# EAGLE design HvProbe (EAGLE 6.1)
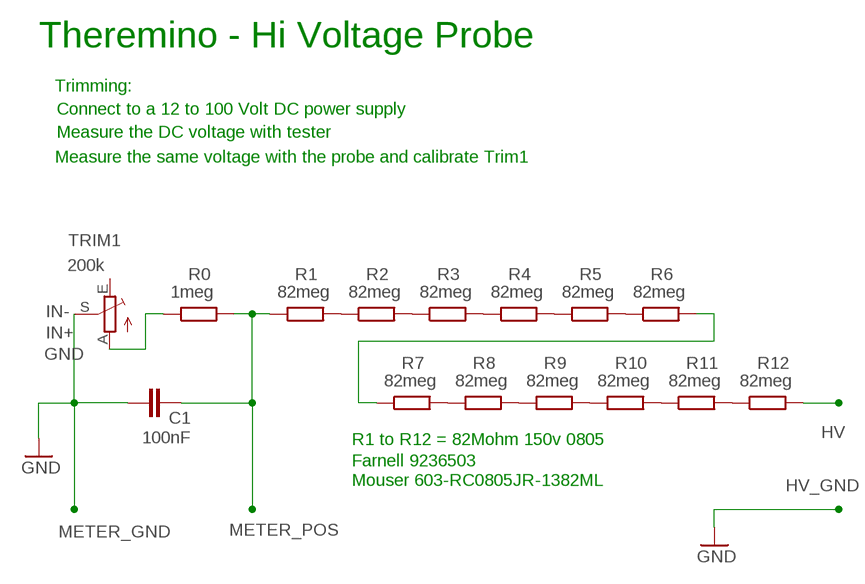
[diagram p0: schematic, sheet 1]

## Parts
C1  100nF  C-EUC0805_L  [C0805_L]
R0  1meg  R-EU_R0805_L  [R0805_L]
R1  82meg  R-EU_R0805_L  [R0805_L]
R2  82meg  R-EU_R0805_L  [R0805_L]
R3  82meg  R-EU_R0805_L  [R0805_L]
R4  82meg  R-EU_R0805_L  [R0805_L]
R5  82meg  R-EU_R0805_L  [R0805_L]
R6  82meg  R-EU_R0805_L  [R0805_L]
R7  82meg  R-EU_R0805_L  [R0805_L]
R8  82meg  R-EU_R0805_L  [R0805_L]
R9  82meg  R-EU_R0805_L  [R0805_L]
R10  82meg  R-EU_R0805_L  [R0805_L]
R11  82meg  R-EU_R0805_L  [R0805_L]
R12  82meg  R-EU_R0805_L  [R0805_L]
TRIM1  200k  TRIMMERTRIM_2H  [TRIM_2H]

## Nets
HV: R12.2
METER_GND: C1.1 TRIM1.S ; supply symbol labelled GND
METER_POS: C1.2 R0.2 R1.1
N$1: R1.2 R2.1
N$2: R2.2 R3.1
N$3: R3.2 R4.1
N$4: R4.2 R5.1
N$5: R5.2 R6.1
N$6: R6.2 R7.1
N$7: R7.2 R8.1
N$8: R8.2 R9.1
N$9: R9.2 R10.1
N$10: R11.2 R12.1
N$11: R10.2 R11.1
N$12: R0.1 TRIM1.A
Unconnected: TRIM1.E

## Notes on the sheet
- Theremino - Hi Voltage Probe
- Trimming:
- Connect to a 12 to 100 Volt DC power supply
- Measure the DC voltage with tester
- Measure the same voltage with the probe and calibrate Trim1
- IN-
- IN+
- GND
- R1 to R12 = 82Mohm 150v 0805
- Farnell 9236503
- Mouser 603-RC0805JR-1382ML

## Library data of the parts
C1 = 00-LIVIO:C-EU: CAPACITOR, European symbol
R0 R1-R12 = 00-LIVIO:R-EU_: RESISTOR, European symbol
TRIM1 = 00-LIVIO:TRIMMER: Horizzontal and Vertical trimmers

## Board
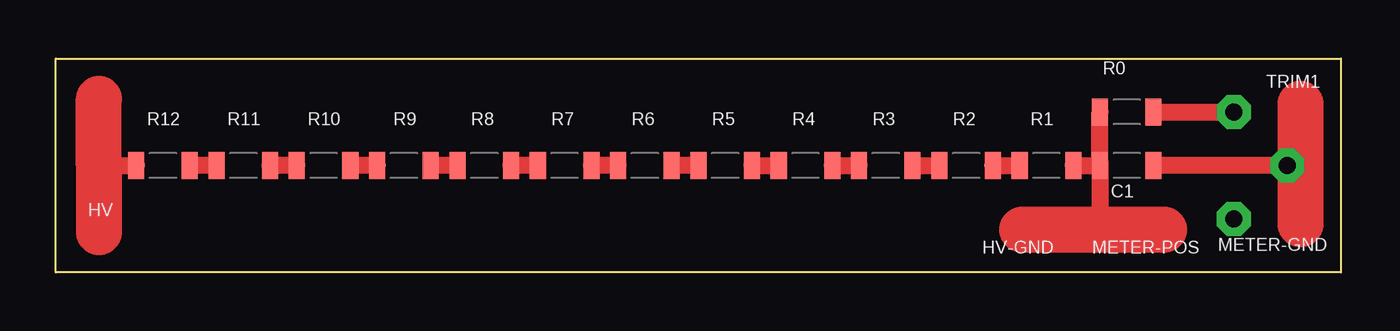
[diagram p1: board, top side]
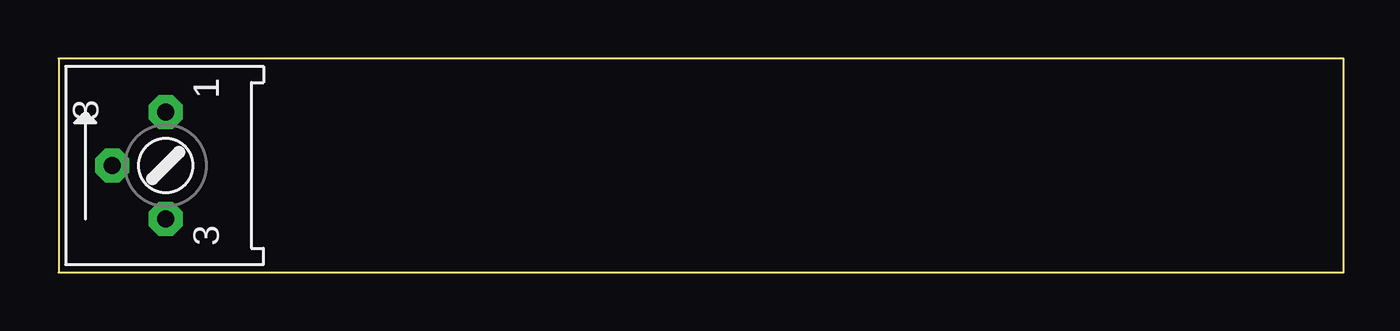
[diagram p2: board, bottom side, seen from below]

Size 60.96 x 10.16 mm. Coordinates in mm from the lower left corner, seen from the top.
Outline: 60.96,0 0,0 0,10.16 60.96,10.16 60.96,0
Copper layers (1*16): Top 0.035mm / dielectric 1.5mm / Bottom 0.035mm
Design rules: minimum track width 10mil, minimum drill 27mil, track to track 27mil, track to pad 27mil, pad to pad 27mil, via to via 27mil, smd to smd 27mil, copper to edge 27mil, drill to drill 8mil, minimum pad ring 5mil, minimum via ring 8mil, stop-mask expansion 4mil, vias tented up to drill 0mil, thermal gap 41mil

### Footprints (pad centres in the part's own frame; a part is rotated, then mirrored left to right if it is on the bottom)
C0805_L = smd 0.762 x 1.27: 1 -1.27,0; 2 1.27,0
R0805_L = smd 0.762 x 1.27: 1 -1.27,0; 2 1.27,0
TRIM_2H = drill 0.8 pad 1.6 octagon: A 2.54,0; E -2.54,0; S 0,2.54

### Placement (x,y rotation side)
C1  50.8,5.08 180 top
R0  50.8,7.62 180 top
R1  46.99,5.08 180 top
R2  43.18,5.08 180 top
R3  39.37,5.08 180 top
R4  35.56,5.08 180 top
R5  31.75,5.08 180 top
R6  27.94,5.08 180 top
R7  24.13,5.08 180 top
R8  20.32,5.08 180 top
R9  16.51,5.08 180 top
R10  12.7,5.08 180 top
R11  8.89,5.08 180 top
R12  5.08,5.08 180 top
TRIM1  55.88,5.08 90 bottom

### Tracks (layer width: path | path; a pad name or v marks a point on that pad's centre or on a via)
HV
  Top 0.813: 2.03,5.08 R12.2
  Top 2.184: 2.03,1.91 2.03,5.08 2.03,8.26
METER_GND
  Top 0.813: C1.1 TRIM1.S 59.05,5.08
  Top 2.184: 59.05,2.29 59.05,5.08 59.05,8
METER_POS
  Top 0.813: R1.1 C1.2 | C1.2 49.53,5.21 R0.2 | C1.2 49.53,2.03
  Top 2.184: 45.85,2.03 49.53,2.03 52.58,2.03
N$1
  Top 0.813: R2.1 R1.2
N$2
  Top 0.813: R3.1 R2.2
N$3
  Top 0.813: R4.1 R3.2
N$4
  Top 0.813: R5.1 R4.2
N$5
  Top 0.813: R5.2 R6.1
N$6
  Top 0.813: R6.2 R7.1
N$7
  Top 0.813: R7.2 R8.1
N$8
  Top 0.813: R8.2 R9.1
N$9
  Top 0.813: R9.2 R10.1
N$10
  Top 0.813: R11.2 R12.1
N$11
  Top 0.813: R10.2 R11.1
N$12
  Top 0.813: R0.1 TRIM1.A

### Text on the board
tNames: HV | HV-GND | METER-POS | METER-GND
